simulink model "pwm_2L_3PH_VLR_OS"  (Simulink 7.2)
settings: Solver=ode3  SolverMode=SingleTasking  StartTime=0.0  StopTime=0.1  FixedStep=10e-6  MaxStep=1e-4  RelTol=1e-3
PreLoadFcn:
  | INIT_PWM_2L

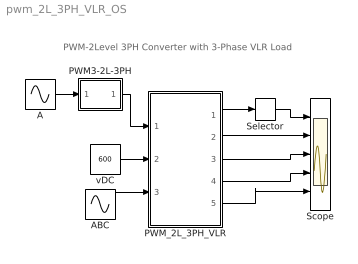
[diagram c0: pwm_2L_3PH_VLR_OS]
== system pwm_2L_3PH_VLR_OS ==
  note: PWM-2Level 3PH Converter with 3-Phase VLR Load
  A : Sin  Amplitude=.7  Frequency=2*pi*50  Phase="[0  -2*pi/3  -4*pi/3]"  SampleTime=0
  ABC : Sin  Amplitude=[0 0 0]  Frequency=2*pi*50  Phase="[0  -2*pi/3 -4*pi/3 ]"  SampleTime=0
  PWM3-2L-3PH : Subsystem  mask(PWM3-2L-3PH){FT=900, PHT=0, DT=1e-6}
      mask prompts: FT "Triangular Frequency"; PHT "Trian. Phase Angle (Degree)"; DT "Dead Time"
      mask help: Pulse Width Modulation for 3 Phase Converter
  PWM_2L_3PH_VLR : Subsystem  mask(pwm_2L_3PH_VLR_OS){RL=0.5, LL=1e-3}
      mask prompts: RL "Load R"; LL "Load L"
      mask help: Open Source 2-Level PWM_3PH Converter with VLR load Input Vector u: u[0]= TD1.gate u[1]= TD2.gate u[2]= TD3.gate u[3]= TD4.gate u[4]= TD5.gate u[5]= TD6.gate u[6]= VDC u[7]= Ea, Phase A Load Voltage u[8]= Eb, Phase B Load Voltage u[9]= Ec, Phase C Load Voltage Output Vector y: y[0]= Va.v, Phase A Output Voltage to middle point y[1]= Vb.V, Phase B Output Voltage to middle point y[2]= Vc.V, Phase C Output Voltage to middle point y[3]= Ia.I, Phase A Output AC Current y[4]= Ib.I, Phase B Output AC Current y[5]= Ic.I, Phase C Output AC Current y[6]= Vab.V, Output AC line Voltage y[7]= T1.I y[8]= D1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
  Scope : Scope  NumInputPorts=5
  Selector : Selector  InputPortWidth=3  IndexOptions=Index vector (dialog)  Indices=[1 ]  OutputSizes=1
  vDC : Constant  Value=600  OutDataType=sfix(16)  OutScaling=2^0
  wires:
  A/1 -> PWM3-2L-3PH/1(In4)
  PWM_2L_3PH_VLR/1(vABC) -> Selector/1
  PWM_2L_3PH_VLR/2(iABC) -> Scope/2
  PWM_2L_3PH_VLR/3(vAB) -> Scope/3
  vDC/1 -> PWM_2L_3PH_VLR/2(vDC)
  PWM3-2L-3PH/1(Out1) -> PWM_2L_3PH_VLR/1(Sw)
  Selector/1 -> Scope/1
  ABC/1 -> PWM_2L_3PH_VLR/3(E_ABC)
  PWM_2L_3PH_VLR/4(iT1,iD1,vT1) -> Scope/4
  PWM_2L_3PH_VLR/5(iDC) -> Scope/5

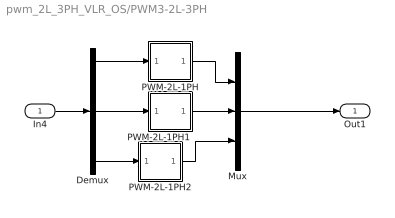
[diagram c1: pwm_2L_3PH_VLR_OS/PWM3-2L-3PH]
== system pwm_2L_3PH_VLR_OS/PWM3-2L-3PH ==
  In4 : Inport
  Demux : Demux  Outputs=3
  Mux : Mux  Inputs=3
  PWM-2L-1PH : Subsystem  mask(PWM-2L-1PH){FT=FT, PHT=PHT, DT=DT}
      mask prompts: FT "Triangular Frequency"; PHT "Trian. Phase Angle (Degree)"; DT "Dead Time"
      mask help: Pulse Width Modulation for 1 Phase Converter
  PWM-2L-1PH1 : Subsystem  mask(PWM-2L-1PH){FT=FT, PHT=PHT, DT=DT}
      mask prompts: FT "Triangular Frequency"; PHT "Trian. Phase Angle (Degree)"; DT "Dead Time"
      mask help: Pulse Width Modulation for 1 Phase Converter
  PWM-2L-1PH2 : Subsystem  mask(PWM-2L-1PH){FT=FT, PHT=PHT, DT=DT}
      mask prompts: FT "Triangular Frequency"; PHT "Trian. Phase Angle (Degree)"; DT "Dead Time"
      mask help: Pulse Width Modulation for 1 Phase Converter
  Out1 : Outport
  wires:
  In4/1 -> Demux/1
  Demux/3 -> PWM-2L-1PH2/1(In1)
  Demux/2 -> PWM-2L-1PH1/1(In1)
  Demux/1 -> PWM-2L-1PH/1(In1)
  PWM-2L-1PH1/1(Out1) -> Mux/2
  PWM-2L-1PH/1(Out1) -> Mux/1
  PWM-2L-1PH2/1(Out1) -> Mux/3
  Mux/1 -> Out1/1

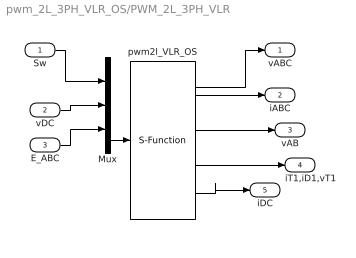
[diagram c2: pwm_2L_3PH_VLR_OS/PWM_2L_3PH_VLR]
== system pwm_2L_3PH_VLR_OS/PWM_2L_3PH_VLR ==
  Sw : Inport  OutDataType=sfix(16)  OutScaling=2^0
  vDC : Inport  Port=2  OutDataType=sfix(16)  OutScaling=2^0
  E_ABC : Inport  Port=3  OutDataType=sfix(16)  OutScaling=2^0
  Mux : Mux  Inputs="[6  1  3]"
  pwm2l_VLR_OS : S-Function  FunctionName=s_pwm_2L_3PH_VLR_OS  Parameters="[RL  LL]"  EnableBusSupport=off
  vABC : Outport  OutDataType=sfix(16)  OutScaling=2^0
  iABC : Outport  Port=2  OutDataType=sfix(16)  OutScaling=2^0
  vAB : Outport  Port=3  OutDataType=sfix(16)  OutScaling=2^0
  iT1,iD1,vT1 : Outport  Port=4  OutDataType=sfix(16)  OutScaling=2^0
  iDC : Outport  Port=5  OutDataType=sfix(16)  OutScaling=2^0
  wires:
  pwm2l_VLR_OS/5 -> iDC/1
  pwm2l_VLR_OS/3 -> vAB/1
  pwm2l_VLR_OS/2 -> iABC/1
  pwm2l_VLR_OS/1 -> vABC/1
  pwm2l_VLR_OS/4 -> iT1,iD1,vT1/1
  E_ABC/1 -> Mux/3
  Mux/1 -> pwm2l_VLR_OS/1
  vDC/1 -> Mux/2
  Sw/1 -> Mux/1

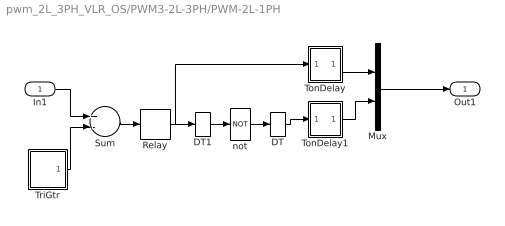
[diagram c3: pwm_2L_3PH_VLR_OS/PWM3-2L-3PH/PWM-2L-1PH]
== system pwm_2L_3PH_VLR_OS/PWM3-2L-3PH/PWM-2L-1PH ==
  In1 : Inport
  DT : DataTypeConversion
  DT1 : DataTypeConversion
  Mux : Mux  Inputs=2
  Relay : Relay
  Sum : Sum  Inputs=+-
  TonDelay : Subsystem  mask(TonDelay){DT=DT}
      mask prompts: DT "Dead Time"
      mask help: Turn on dead time to protect against short circuit of the converter leg
  TonDelay1 : Subsystem  mask(TonDelay){DT=DT}
      mask prompts: DT "Dead Time"
      mask help: Turn on dead time to protect against short circuit of the converter leg
  TriGtr : Subsystem  mask(TriGtr){T=1/FT, Td=PHT/FT/360}
      mask prompts: T "Period Time"; Td "Time Delay"
      mask help: Triangular Wave Generator with variable time delay
  not : Logic  Operator=NOT  Inputs=1
  Out1 : Outport  InitialOutput=0
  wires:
  Mux/1 -> Out1/1
  TonDelay/1(s1d) -> Mux/1
  Relay/1 -> TonDelay/1(s1), DT1/1
  TonDelay1/1(s1d) -> Mux/2
  not/1 -> DT/1
  Sum/1 -> Relay/1
  TriGtr/1(O) -> Sum/2
  In1/1 -> Sum/1
  DT/1 -> TonDelay1/1(s1)
  DT1/1 -> not/1

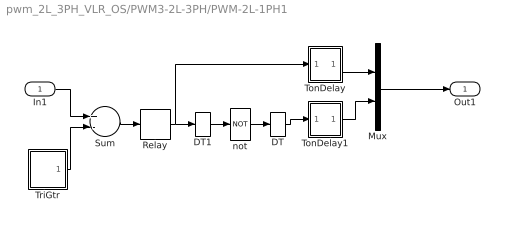
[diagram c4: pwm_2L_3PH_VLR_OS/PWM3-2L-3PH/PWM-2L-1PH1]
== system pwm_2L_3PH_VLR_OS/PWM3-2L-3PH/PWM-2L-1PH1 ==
  In1 : Inport
  DT : DataTypeConversion
  DT1 : DataTypeConversion
  Mux : Mux  Inputs=2
  Relay : Relay
  Sum : Sum  Inputs=+-
  TonDelay : Subsystem  mask(TonDelay){DT=DT}
      mask prompts: DT "Dead Time"
      mask help: Turn on dead time to protect against short circuit of the converter leg
  TonDelay1 : Subsystem  mask(TonDelay){DT=DT}
      mask prompts: DT "Dead Time"
      mask help: Turn on dead time to protect against short circuit of the converter leg
  TriGtr : Subsystem  mask(TriGtr){T=1/FT, Td=PHT/FT/360}
      mask prompts: T "Period Time"; Td "Time Delay"
      mask help: Triangular Wave Generator with variable time delay
  not : Logic  Operator=NOT  Inputs=1
  Out1 : Outport  InitialOutput=0
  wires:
  DT1/1 -> not/1
  DT/1 -> TonDelay1/1(s1)
  In1/1 -> Sum/1
  TriGtr/1(O) -> Sum/2
  Sum/1 -> Relay/1
  not/1 -> DT/1
  TonDelay1/1(s1d) -> Mux/2
  Relay/1 -> DT1/1, TonDelay/1(s1)
  TonDelay/1(s1d) -> Mux/1
  Mux/1 -> Out1/1

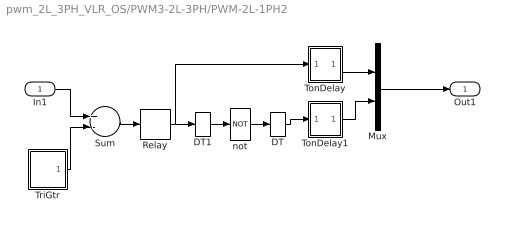
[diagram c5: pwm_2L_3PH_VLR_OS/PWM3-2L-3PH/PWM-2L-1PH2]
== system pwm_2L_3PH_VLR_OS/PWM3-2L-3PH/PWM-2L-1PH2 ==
  In1 : Inport
  DT : DataTypeConversion
  DT1 : DataTypeConversion
  Mux : Mux  Inputs=2
  Relay : Relay
  Sum : Sum  Inputs=+-
  TonDelay : Subsystem  mask(TonDelay){DT=DT}
      mask prompts: DT "Dead Time"
      mask help: Turn on dead time to protect against short circuit of the converter leg
  TonDelay1 : Subsystem  mask(TonDelay){DT=DT}
      mask prompts: DT "Dead Time"
      mask help: Turn on dead time to protect against short circuit of the converter leg
  TriGtr : Subsystem  mask(TriGtr){T=1/FT, Td=PHT/FT/360}
      mask prompts: T "Period Time"; Td "Time Delay"
      mask help: Triangular Wave Generator with variable time delay
  not : Logic  Operator=NOT  Inputs=1
  Out1 : Outport  InitialOutput=0
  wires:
  Mux/1 -> Out1/1
  TonDelay/1(s1d) -> Mux/1
  Relay/1 -> TonDelay/1(s1), DT1/1
  TonDelay1/1(s1d) -> Mux/2
  not/1 -> DT/1
  Sum/1 -> Relay/1
  TriGtr/1(O) -> Sum/2
  In1/1 -> Sum/1
  DT/1 -> TonDelay1/1(s1)
  DT1/1 -> not/1

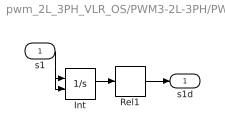
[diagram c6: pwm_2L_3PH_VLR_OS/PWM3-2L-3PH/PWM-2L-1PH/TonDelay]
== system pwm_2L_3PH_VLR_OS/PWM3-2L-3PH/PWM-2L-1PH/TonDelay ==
  s1 : Inport
  Int : Integrator  ExternalReset=falling
  Rel1 : Relay  OnSwitchValue=DT
  s1d : Outport  InitialOutput=0
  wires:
  Rel1/1 -> s1d/1
  s1/1 -> Int/1, Int/2
  Int/1 -> Rel1/1

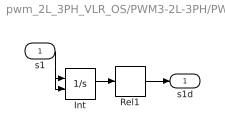
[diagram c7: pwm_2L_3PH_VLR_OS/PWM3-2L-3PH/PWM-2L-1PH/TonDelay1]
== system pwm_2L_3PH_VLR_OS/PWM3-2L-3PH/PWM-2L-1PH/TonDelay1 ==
  s1 : Inport
  Int : Integrator  ExternalReset=falling
  Rel1 : Relay  OnSwitchValue=DT
  s1d : Outport  InitialOutput=0
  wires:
  Rel1/1 -> s1d/1
  s1/1 -> Int/1, Int/2
  Int/1 -> Rel1/1

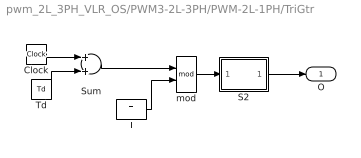
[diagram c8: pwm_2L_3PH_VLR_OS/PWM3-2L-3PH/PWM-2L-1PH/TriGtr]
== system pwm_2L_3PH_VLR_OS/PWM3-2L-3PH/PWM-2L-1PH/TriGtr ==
  Clock : Clock
  S2 : Subsystem
  Sum : Sum
  T : Constant  Value=T
  Td : Constant  Value=Td
  mod : Math  Operator=mod
  O : Outport  InitialOutput=0
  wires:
  Td/1 -> Sum/2
  Sum/1 -> mod/1
  T/1 -> mod/2
  Clock/1 -> Sum/1
  S2/1(O1) -> O/1
  mod/1 -> S2/1(I1)

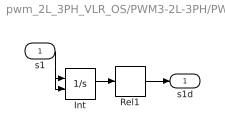
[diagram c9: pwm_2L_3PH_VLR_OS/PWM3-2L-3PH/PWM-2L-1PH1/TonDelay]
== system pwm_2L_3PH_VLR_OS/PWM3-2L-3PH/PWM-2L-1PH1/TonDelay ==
  s1 : Inport
  Int : Integrator  ExternalReset=falling
  Rel1 : Relay  OnSwitchValue=DT
  s1d : Outport  InitialOutput=0
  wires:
  Int/1 -> Rel1/1
  s1/1 -> Int/2, Int/1
  Rel1/1 -> s1d/1

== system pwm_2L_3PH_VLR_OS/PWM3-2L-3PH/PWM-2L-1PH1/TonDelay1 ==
  s1 : Inport
  Int : Integrator  ExternalReset=falling
  Rel1 : Relay  OnSwitchValue=DT
  s1d : Outport  InitialOutput=0
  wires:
  Int/1 -> Rel1/1
  s1/1 -> Int/2, Int/1
  Rel1/1 -> s1d/1

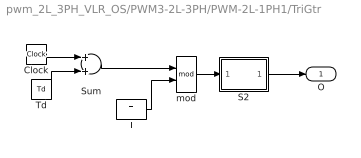
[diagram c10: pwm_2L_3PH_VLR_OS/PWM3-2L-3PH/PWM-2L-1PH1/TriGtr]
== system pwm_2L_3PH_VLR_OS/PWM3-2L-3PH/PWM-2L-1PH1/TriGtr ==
  Clock : Clock
  S2 : Subsystem
  Sum : Sum
  T : Constant  Value=T
  Td : Constant  Value=Td
  mod : Math  Operator=mod
  O : Outport  InitialOutput=0
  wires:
  mod/1 -> S2/1(I1)
  S2/1(O1) -> O/1
  Clock/1 -> Sum/1
  T/1 -> mod/2
  Sum/1 -> mod/1
  Td/1 -> Sum/2

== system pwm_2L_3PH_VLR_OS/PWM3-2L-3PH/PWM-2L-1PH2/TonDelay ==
  s1 : Inport
  Int : Integrator  ExternalReset=falling
  Rel1 : Relay  OnSwitchValue=DT
  s1d : Outport  InitialOutput=0
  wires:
  Rel1/1 -> s1d/1
  s1/1 -> Int/1, Int/2
  Int/1 -> Rel1/1

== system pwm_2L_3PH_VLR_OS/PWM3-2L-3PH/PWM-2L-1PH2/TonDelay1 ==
  s1 : Inport
  Int : Integrator  ExternalReset=falling
  Rel1 : Relay  OnSwitchValue=DT
  s1d : Outport  InitialOutput=0
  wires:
  Rel1/1 -> s1d/1
  s1/1 -> Int/1, Int/2
  Int/1 -> Rel1/1

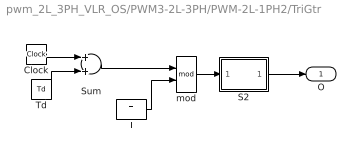
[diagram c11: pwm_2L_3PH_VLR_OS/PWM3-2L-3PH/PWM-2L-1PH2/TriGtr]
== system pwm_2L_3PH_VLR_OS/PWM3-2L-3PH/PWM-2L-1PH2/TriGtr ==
  Clock : Clock
  S2 : Subsystem
  Sum : Sum
  T : Constant  Value=T
  Td : Constant  Value=Td
  mod : Math  Operator=mod
  O : Outport  InitialOutput=0
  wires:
  Td/1 -> Sum/2
  Sum/1 -> mod/1
  T/1 -> mod/2
  Clock/1 -> Sum/1
  S2/1(O1) -> O/1
  mod/1 -> S2/1(I1)

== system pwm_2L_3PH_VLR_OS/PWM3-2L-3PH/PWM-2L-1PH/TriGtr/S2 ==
  I1 : Inport
  Fcn : Fcn  Expr="(u* (u <=T/4) * 4/T)   +  (  (u > T/4) && ( u <=3*T/4) )* ( 1 - (u-T/4) *4/T )   +  ( (u > 3*T/4)&& (u<=T)) * ( ((u -3*T/4)* 4/T )-1 )"
  O1 : Outport
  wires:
  I1/1 -> Fcn/1
  Fcn/1 -> O1/1

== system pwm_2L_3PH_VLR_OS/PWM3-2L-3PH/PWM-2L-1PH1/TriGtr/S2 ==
  I1 : Inport
  Fcn : Fcn  Expr="(u* (u <=T/4) * 4/T)   +  (  (u > T/4) && ( u <=3*T/4) )* ( 1 - (u-T/4) *4/T )   +  ( (u > 3*T/4)&& (u<=T)) * ( ((u -3*T/4)* 4/T )-1 )"
  O1 : Outport
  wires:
  Fcn/1 -> O1/1
  I1/1 -> Fcn/1

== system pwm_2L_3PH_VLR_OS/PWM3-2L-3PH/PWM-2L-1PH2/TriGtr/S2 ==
  I1 : Inport
  Fcn : Fcn  Expr="(u* (u <=T/4) * 4/T)   +  (  (u > T/4) && ( u <=3*T/4) )* ( 1 - (u-T/4) *4/T )   +  ( (u > 3*T/4)&& (u<=T)) * ( ((u -3*T/4)* 4/T )-1 )"
  O1 : Outport
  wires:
  I1/1 -> Fcn/1
  Fcn/1 -> O1/1
